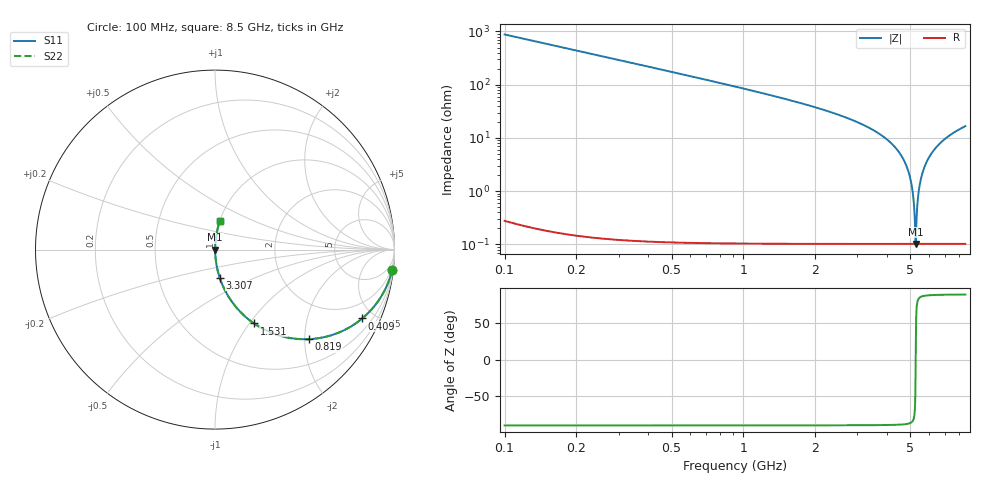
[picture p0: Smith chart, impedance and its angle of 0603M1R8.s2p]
! Created Wed Apr 18 13:52:57 2012
# hz S ma R 50
! 2 Port Network Data from SP1.SP block
! freq  magS11  angS11  magS21  angS21  magS12  angS12  magS22  angS22
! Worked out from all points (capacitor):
!   8401 points, 100 MHz to 8.5 GHz, reference 50 ohm
!   read as one part in series: C = 1.81 pF near 142 MHz
!   lowest |Z| = 102 mohm at 5.263 GHz (marker M1)
!   series resonance near 5.263 GHz, so ESL is about 510 pH
!   S11 on the Smith chart (normalised r, x): 100 MHz: 1, -18; 409 MHz: 1.00, -4.27; 819 MHz: 1.00, -2.10; 1.531 GHz: 1.00, -1.05; 3.307 GHz: 1.00, -0.32; 8.5 GHz: 1.00, +0.33
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1e8  0.9936 -6.5  0.113 83.5  0.113 83.5  0.9936 -6.5
2.38e8  0.965 -15.2  0.2617 74.8  0.2617 74.8  0.965 -15.2
4.09e8  0.9056 -25.1  0.4238 64.9  0.4238 64.9  0.9056 -25.1
8.19e8  0.723 -43.6  0.6901 46.3  0.6901 46.3  0.723 -43.6
1.5e9  0.4738 -61.6  0.8797 28.3  0.8797 28.3  0.4738 -61.6
1.531e9  0.465 -62.2  0.8844 27.7  0.8844 27.7  0.465 -62.2
2.9e9  0.2064 -77.8  0.9775 11.9  0.9775 11.9  0.2064 -77.8
3.307e9  0.1587 -80.5  0.9863 9.1  0.9863 9.1  0.1587 -80.5
4.3e9  0.06778 -85.3  0.9967 3.9  0.9967 3.9  0.06778 -85.3
4.72e9  0.03641 -86.3  0.9983 2.1  0.9983 2.1  0.03641 -86.3
4.994e9  0.01753 -85.7  0.9988 1.0  0.9988 1.0  0.01753 -85.7
5.144e9  0.007682 -81.9  0.999 0.4  0.999 0.4  0.007682 -81.9
5.189e9  0.004813 -77.5  0.999 0.3  0.999 0.3  0.004813 -77.5
5.238e9  0.001867 -56.8  0.999 0.1  0.999 0.1  0.001867 -56.8
5.263e9  0.00102 1.5  0.999 -0.0  0.999 -0.0  0.00102 1.5
5.289e9  0.001959 58.6  0.999 -0.1  0.999 -0.1  0.001959 58.6
5.354e9  0.005844 79.6  0.999 -0.3  0.999 -0.3  0.005844 79.6
5.42e9  0.009901 83.5  0.9989 -0.6  0.9989 -0.6  0.009901 83.5
5.7e9  0.02672 86.3  0.9986 -1.5  0.9986 -1.5  0.02672 86.3
6.236e9  0.05691 85.7  0.9974 -3.3  0.9974 -3.3  0.05691 85.7
7.1e9  0.1011 83.6  0.9939 -5.8  0.9939 -5.8  0.1011 83.6
8.5e9  0.1643 80.2  0.9854 -9.5  0.9854 -9.5  0.1643 80.2
